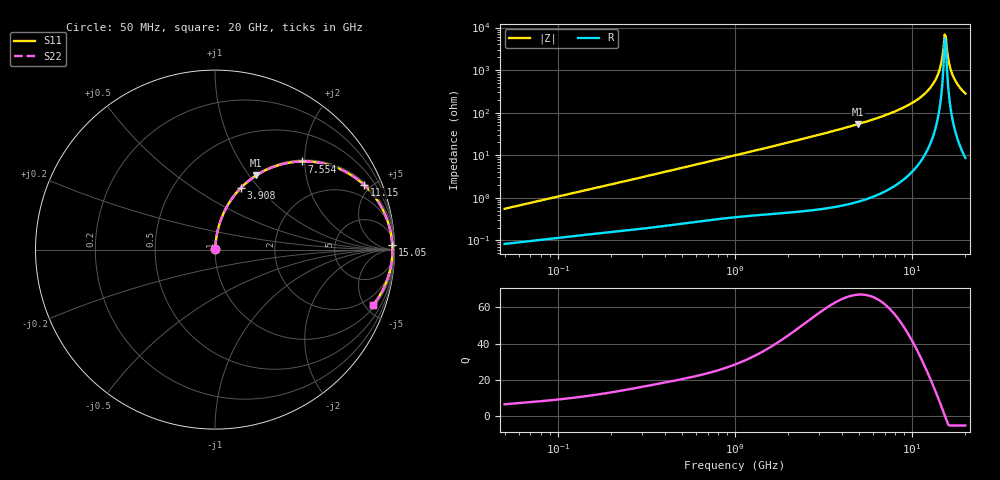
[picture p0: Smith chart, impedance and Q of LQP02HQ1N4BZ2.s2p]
!Murata Part Number: LQP02HQ1N4BZ2
!These Parameters are Measured in Series Mode Connection
!  o--[Z]--o
!Port1  Port2
!  o-------o
!Freq. Start=50[MHz] Stop=20[GHz], 401[Steps]
# Hz S RI R 50
!Freq.(Hz) S11(Real) S11(Imag) S21(Real) S21(Imag) S12(Real) S12(Imag) S22(Real) S22(Imag)
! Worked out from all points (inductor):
!   401 points, 50 MHz to 20 GHz, reference 50 ohm
!   read as one part in series: L = 1.72 nH near 51.52 MHz
!   highest Q = 66.8 at 4.967 GHz (marker M1), where L = 1.73 nH
!   self-resonance near 15.27 GHz
!   S11 on the Smith chart (normalised r, x): 50 MHz: 1.00, +0.01; 3.908 GHz: 1.01, +0.82; 7.554 GHz: 1.03, +1.94; 11.15 GHz: 1.14, +4.58; 15.05 GHz: 26, +60; 20 GHz: 1.17, -5.62
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5e7  0.000853 0.00545  0.9991 -0.00545  0.9991 -0.00545  0.000853 0.00545
1.364002e8  0.00152 0.0142  0.9985 -0.0142  0.9985 -0.0142  0.00152 0.0142
3.721004e8  0.0035 0.0374  0.9965 -0.0374  0.9965 -0.0374  0.0035 0.0374
1e9  0.0131 0.0976  0.9869 -0.0976  0.9869 -0.0976  0.0131 0.0976
2.728004e9  0.0745 0.2534  0.9255 -0.2534  0.9255 -0.2534  0.0745 0.2534
3.908127e9  0.1464 0.3458  0.8536 -0.3458  0.8536 -0.3458  0.1464 0.3458
4.966507e9  0.2297 0.4133  0.7703 -0.4133  0.7703 -0.4133  0.2297 0.4133
7.442007e9  0.4736 0.4909  0.5264 -0.4909  0.5264 -0.4909  0.4736 0.4909
7.554318e9  0.4855 0.4913  0.5145 -0.4913  0.5145 -0.4913  0.4855 0.4913
9.316812e9  0.6698 0.4597  0.3302 -0.4597  0.3302 -0.4597  0.6698 0.4597
1.115139e10  0.8328 0.3581  0.1672 -0.3581  0.1672 -0.3581  0.8328 0.3581
1.257102e10  0.9219 0.2461  0.0781 -0.2461  0.0781 -0.2461  0.9219 0.2461
1.375312e10  0.9671 0.1422  0.0329 -0.1422  0.0329 -0.1422  0.9671 0.1422
1.438523e10  0.9807 0.0859  0.0193 -0.0859  0.0193 -0.0859  0.9807 0.0859
1.504638e10  0.9876 0.0279  0.0124 -0.0279  0.0124 -0.0279  0.9876 0.0279
1.527346e10  0.9883 0.0084  0.0117 -0.0084  0.0117 -0.0084  0.9883 0.0084
1.550395e10  0.9884 -0.0111  0.0116 0.0111  0.0116 0.0111  0.9884 -0.0111
1.573793e10  0.9876 -0.0306  0.0124 0.0306  0.0124 0.0306  0.9876 -0.0306
1.646126e10  0.9807 -0.0886  0.0193 0.0886  0.0193 0.0886  0.9807 -0.0886
1.747767e10  0.9611 -0.1633  0.0389 0.1633  0.0389 0.1633  0.9611 -0.1633
1.855685e10  0.9308 -0.2327  0.0692 0.2327  0.0692 0.2327  0.9308 -0.2327
2e10  0.8804 -0.3095  0.1196 0.3095  0.1196 0.3095  0.8804 -0.3095
